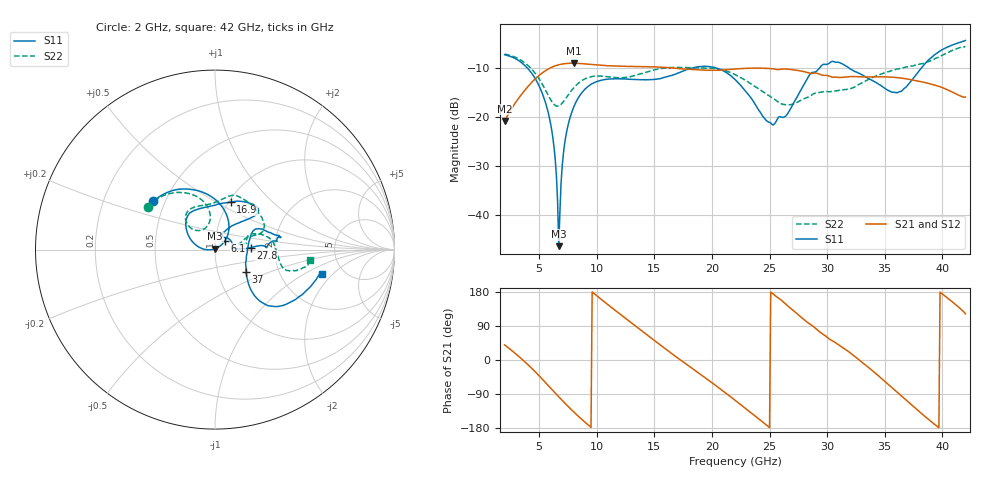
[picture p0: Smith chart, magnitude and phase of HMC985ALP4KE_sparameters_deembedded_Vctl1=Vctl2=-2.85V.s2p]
!s2p File: Measurements: S11, S21, S12, S22
# GHz S dB R 50.0
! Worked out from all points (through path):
!   401 points, 2 GHz to 42 GHz, reference 50 ohm
!   highest |S21| = -8.94 dB at 8 GHz (marker M1); lowest = -20.7 dB at 2 GHz (marker M2)
!   lowest |S11| = -46.3 dB at 6.7 GHz (marker M3), VSWR 1.01, Z = 50 + j0.482 ohm
!   |S11| at or under -10 dB: 4.007 GHz to 18.16 GHz (14.15 GHz wide, 128 % of centre); 20.48 GHz to 29.3 GHz (8.825 GHz wide, 35.5 % of centre); 31.95 GHz to 38.14 GHz (6.194 GHz wide, 17.7 % of centre)
!   |S22| runs from -17.7 to -5.5 dB; largest |S21 - S12| = 0.0004
!   S11 on the Smith chart (normalised r, x): 2 GHz: 0.43, +0.29; 6.1 GHz: 1.11, +0.11; 16.9 GHz: 1.02, +0.59; 27.8 GHz: 1.49, +0.03; 37 GHz: 1.36, -0.36; 42 GHz: 3.44, -1.50
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2  -7.20 141.7  -20.75 39.8  -20.75 39.8  -7.06 147.4
4.6  -11.85 84.0  -12.27 -29.4  -12.28 -29.4  -10.82 105.2
6.1  -22.75 41.4  -9.75 -77.6  -9.75 -77.6  -16.78 104.7
6.7  -46.34 89.9  -9.25 -97.1  -9.25 -97.1  -17.66 122.6
6.9  -33.46 -178.6  -9.14 -103.5  -9.15 -103.5  -17.33 128.4
7.3  -24.04 177.6  -9.00 -116.1  -9.01 -116.1  -16.17 135.8
8  -17.88 162.1  -8.94 -137.1  -8.94 -137.1  -13.97 138.0
8.7  -14.98 149.4  -9.02 -156.7  -9.03 -156.8  -12.50 133.8
12.3  -12.13 118.6  -9.56 114.5  -9.56 114.5  -11.88 97.6
15.4  -12.15 90.5  -9.73 42.3  -9.73 42.3  -10.09 73.8
16.9  -11.11 71.8  -9.97 8.0  -9.97 8.0  -9.79 66.8
19.6  -9.57 44.0  -10.39 -51.0  -10.39 -51.0  -9.96 40.0
22  -12.24 43.3  -10.12 -106.1  -10.12 -106.1  -11.25 19.9
25.2  -21.43 57.4  -10.06 176.8  -10.06 176.8  -15.99 17.1
27.8  -14.06 3.0  -10.56 111.4  -10.56 111.4  -16.42 10.6
28.7  -10.82 2.2  -11.01 90.9  -11.01 90.9  -15.35 11.2
30.5  -8.55 10.6  -11.80 49.8  -11.81 49.7  -14.62 17.6
32.4  -10.63 21.7  -11.67 9.3  -11.67 9.3  -13.77 23.0
35.4  -14.60 6.6  -11.75 -66.9  -11.75 -66.9  -10.62 14.5
37  -13.41 -36.0  -12.18 -109.7  -12.18 -109.7  -9.65 6.0
39.6  -6.76 -43.8  -13.59 -176.3  -13.59 -176.3  -7.76 -15.9
42  -4.28 -12.9  -15.86 121.7  -15.87 121.6  -5.50 -6.5
